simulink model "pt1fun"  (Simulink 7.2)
settings: Solver=ode45  StartTime=0.0  StopTime=10.0  RelTol=1e-3

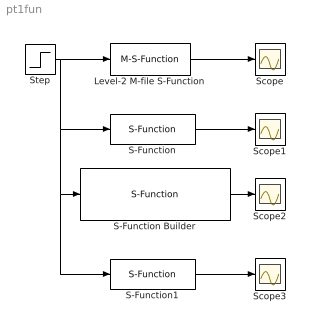
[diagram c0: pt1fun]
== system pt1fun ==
  Level-2 M-file S-Function : M-S-Function  FunctionName=pt1sfun_m2  Parameters=T
  S-Function : S-Function  FunctionName=pt1sfun_c  Parameters=T  EnableBusSupport=off
  S-Function Builder : S-Function  FunctionName=pt1sfun_csfb  Parameters=T  SFunctionModules=pt1sfun_csfb_wrapper  WizardData=DataTag0  EnableBusSupport=off
  S-Function1 : S-Function  FunctionName=pt1sfun_m  Parameters=T  EnableBusSupport=off
  Scope{,1..3} (4 alike) : Scope
  Step : Step  SampleTime=0
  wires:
  Step/1 -> S-Function/1, S-Function1/1, S-Function Builder/1, Level-2 M-file S-Function/1
  Level-2 M-file S-Function/1 -> Scope/1
  S-Function/1 -> Scope1/1
  S-Function1/1 -> Scope3/1
  S-Function Builder/1 -> Scope2/1
